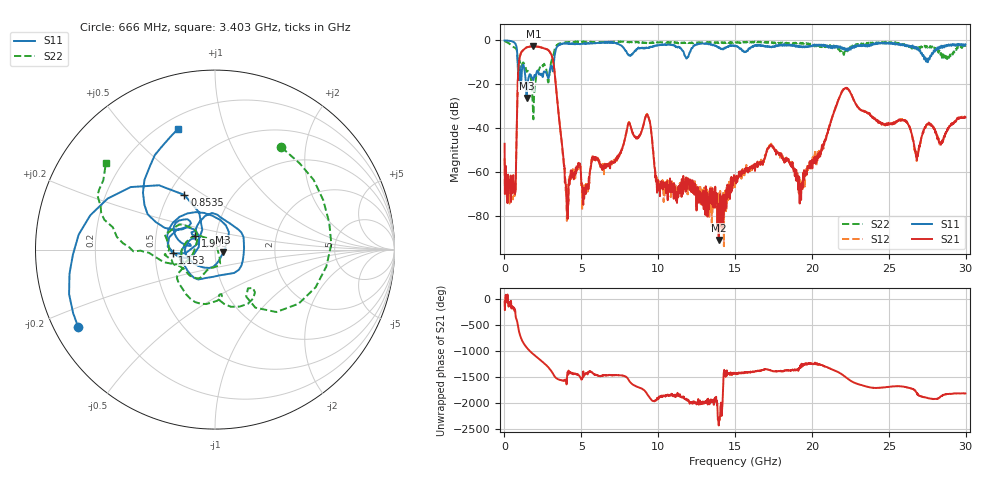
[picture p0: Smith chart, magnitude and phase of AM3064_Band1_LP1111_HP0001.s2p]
# Hz S DB R 50.0
!freq dBS11 angS11 dBS21 angS21 dBS12 angS12 dBS22 angS22
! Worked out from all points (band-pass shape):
!   1600 points, 10 MHz to 29.98 GHz, reference 50 ohm
!   highest |S21| = -2.63 dB at 1.884 GHz (marker M1); lowest = -91.0 dB at 13.94 GHz (marker M2)
!   |S21| within 3 dB of the highest: 1.081 GHz to 2.987 GHz (1.906 GHz wide, 93.7 % of centre)
!   lowest |S11| = -26.3 dB at 1.435 GHz (marker M3), VSWR 1.10, Z = 54.8 - j1.74 ohm
!   |S11| at or under -10 dB: 857.7 MHz to 3.219 GHz (2.361 GHz wide, 116 % of centre)
!   |S22| runs from -36.0 to -0.2 dB; largest |S21 - S12| = 0.013
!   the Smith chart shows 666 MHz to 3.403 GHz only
!   S11 on the Smith chart (normalised r, x): 666 MHz: 0.07, -0.26; 853.5 MHz: 0.60, +0.42; 1.153 GHz: 0.62, -0.02; 1.903 GHz: 0.79, +0.12; 3.403 GHz: 0.26, +0.71
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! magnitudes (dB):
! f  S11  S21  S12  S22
! 10 MHz  0.0  -47.1  -53.8  -0.2
! 666 MHz  -1.1  -65.7  -70.9  -3.4
! 853.5 MHz  -9.1  -22.2  -22.1  -8.1
! 1.153 GHz  -12.5  -4.9  -4.9  -10.9
! 1.435 GHz  -26.3  -3.2  -3.2  -14.2
! 1.884 GHz  -17.9  -2.6  -2.7  -36.0
! 1.903 GHz  -17.4  -2.7  -2.6  -29.7
! 2.99 GHz  -12.3  -5.7  -5.7  -11.8
! 3.403 GHz  -3.0  -25.0  -25.0  -2.2
! 4.021 GHz  -1.4  -69.5  -70.9  -1.0
! 5.015 GHz  -1.6  -65.0  -66.2  -0.5
! 9.269 GHz  -3.3  -33.7  -33.5  -1.2
! 10 GHz  -2.2  -63.7  -67.1  -0.9
! 13.94 GHz  -3.1  -91.0  -75.6  -1.0
! 15 GHz  -2.6  -63.8  -64.7  -1.1
! 17.27 GHz  -3.1  -48.2  -48.1  -1.1
! 19.24 GHz  -2.9  -65.6  -66.9  -1.4
! 19.99 GHz  -2.7  -55.4  -54.7  -1.7
! 22.13 GHz  -4.1  -22.1  -22.0  -5.3
! 25 GHz  -1.0  -37.9  -38.4  -1.1
! 26.83 GHz  -3.9  -54.6  -54.1  -3.2
! 29.98 GHz  -1.8  -35.1  -35.1  -2.9
